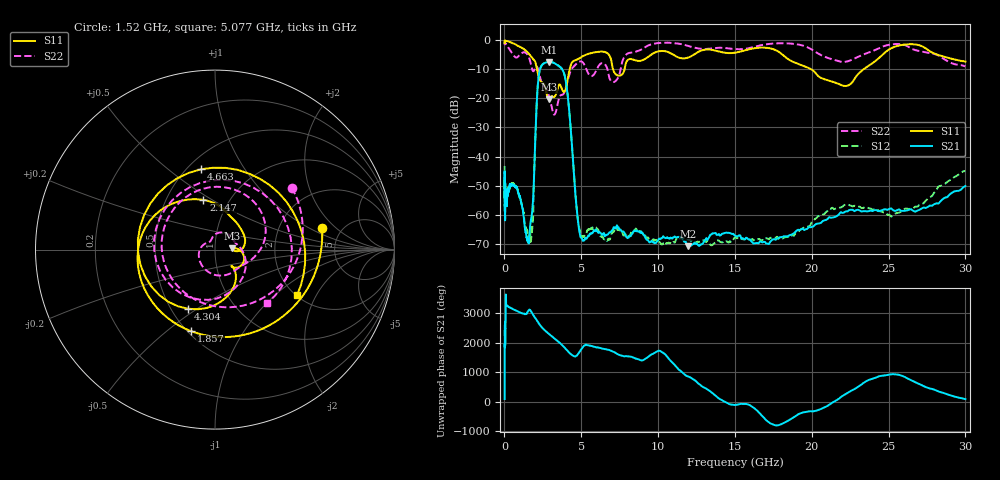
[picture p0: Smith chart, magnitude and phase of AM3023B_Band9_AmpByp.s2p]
# Hz S DB R 50.0
!freq dBS11 angS11 dBS21 angS21 dBS12 angS12 dBS22 angS22
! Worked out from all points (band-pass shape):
!   1601 points, 10 MHz to 30 GHz, reference 50 ohm
!   highest |S21| = -7.58 dB at 2.928 GHz (marker M1); lowest = -70.8 dB at 11.95 GHz (marker M2)
!   |S21| within 3 dB of the highest: 2.289 GHz to 3.811 GHz (1.521 GHz wide, 49.9 % of centre)
!   lowest |S11| = -20.4 dB at 2.899 GHz (marker M3), VSWR 1.21, Z = 60.5 + j0.872 ohm
!   |S11| at or under -10 dB: 2.108 GHz to 4.246 GHz (2.138 GHz wide, 67.3 % of centre); 7.06 GHz to 7.819 GHz (759.2 MHz wide, 10.2 % of centre); 19.94 GHz to 23.39 GHz (3.451 GHz wide, 15.9 % of centre)
!   |S22| runs from -25.6 to -0.9 dB; largest |S21 - S12| = 0.0089
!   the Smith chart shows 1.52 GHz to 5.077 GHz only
!   S11 on the Smith chart (normalised r, x): 1.52 GHz: 3.54, +1.37; 1.857 GHz: 0.52, -0.61; 2.147 GHz: 0.76, +0.46; 4.304 GHz: 0.61, -0.46; 4.663 GHz: 0.58, +0.66; 5.077 GHz: 2.04, -1.41
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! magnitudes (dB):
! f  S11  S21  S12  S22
! 10 MHz  -0.4  -53.8  -43.6  -0.9
! 12.09 MHz  -0.8  -45.8  -49.0  -1.3
! 38.04 MHz  -0.2  -60.6  -59.4  -0.9
! 49.1 MHz  -0.3  -49.7  -50.7  -1.1
! 144.7 MHz  -0.4  -54.4  -53.5  -1.7
! 547.7 MHz  -1.2  -49.8  -49.4  -5.1
! 1.52 GHz  -4.3  -69.1  -66.5  -5.2
! 1.857 GHz  -6.5  -55.3  -61.4  -10.7
! 2.084 GHz  -9.4  -23.5  -23.4  -9.1
! 2.147 GHz  -10.9  -17.3  -17.3  -9.5
! 2.899 GHz  -20.4  -7.6  -7.6  -19.2
! 2.928 GHz  -20.3  -7.6  -7.6  -19.7
! 3.837 GHz  -17.7  -10.9  -10.9  -18.6
! 4.304 GHz  -8.8  -29.9  -29.9  -10.7
! 4.663 GHz  -6.9  -56.2  -55.7  -8.3
! 5.077 GHz  -5.6  -68.7  -67.2  -7.6
! 7.926 GHz  -7.7  -67.6  -67.4  -5.0
! 11.95 GHz  -6.1  -70.8  -68.6  -2.0
! 18.37 GHz  -6.2  -67.4  -67.6  -1.2
! 21.78 GHz  -15.1  -59.8  -57.6  -7.3
! 25.95 GHz  -1.7  -58.7  -58.2  -1.6
! 30 GHz  -7.4  -50.1  -45.0  -9.1
